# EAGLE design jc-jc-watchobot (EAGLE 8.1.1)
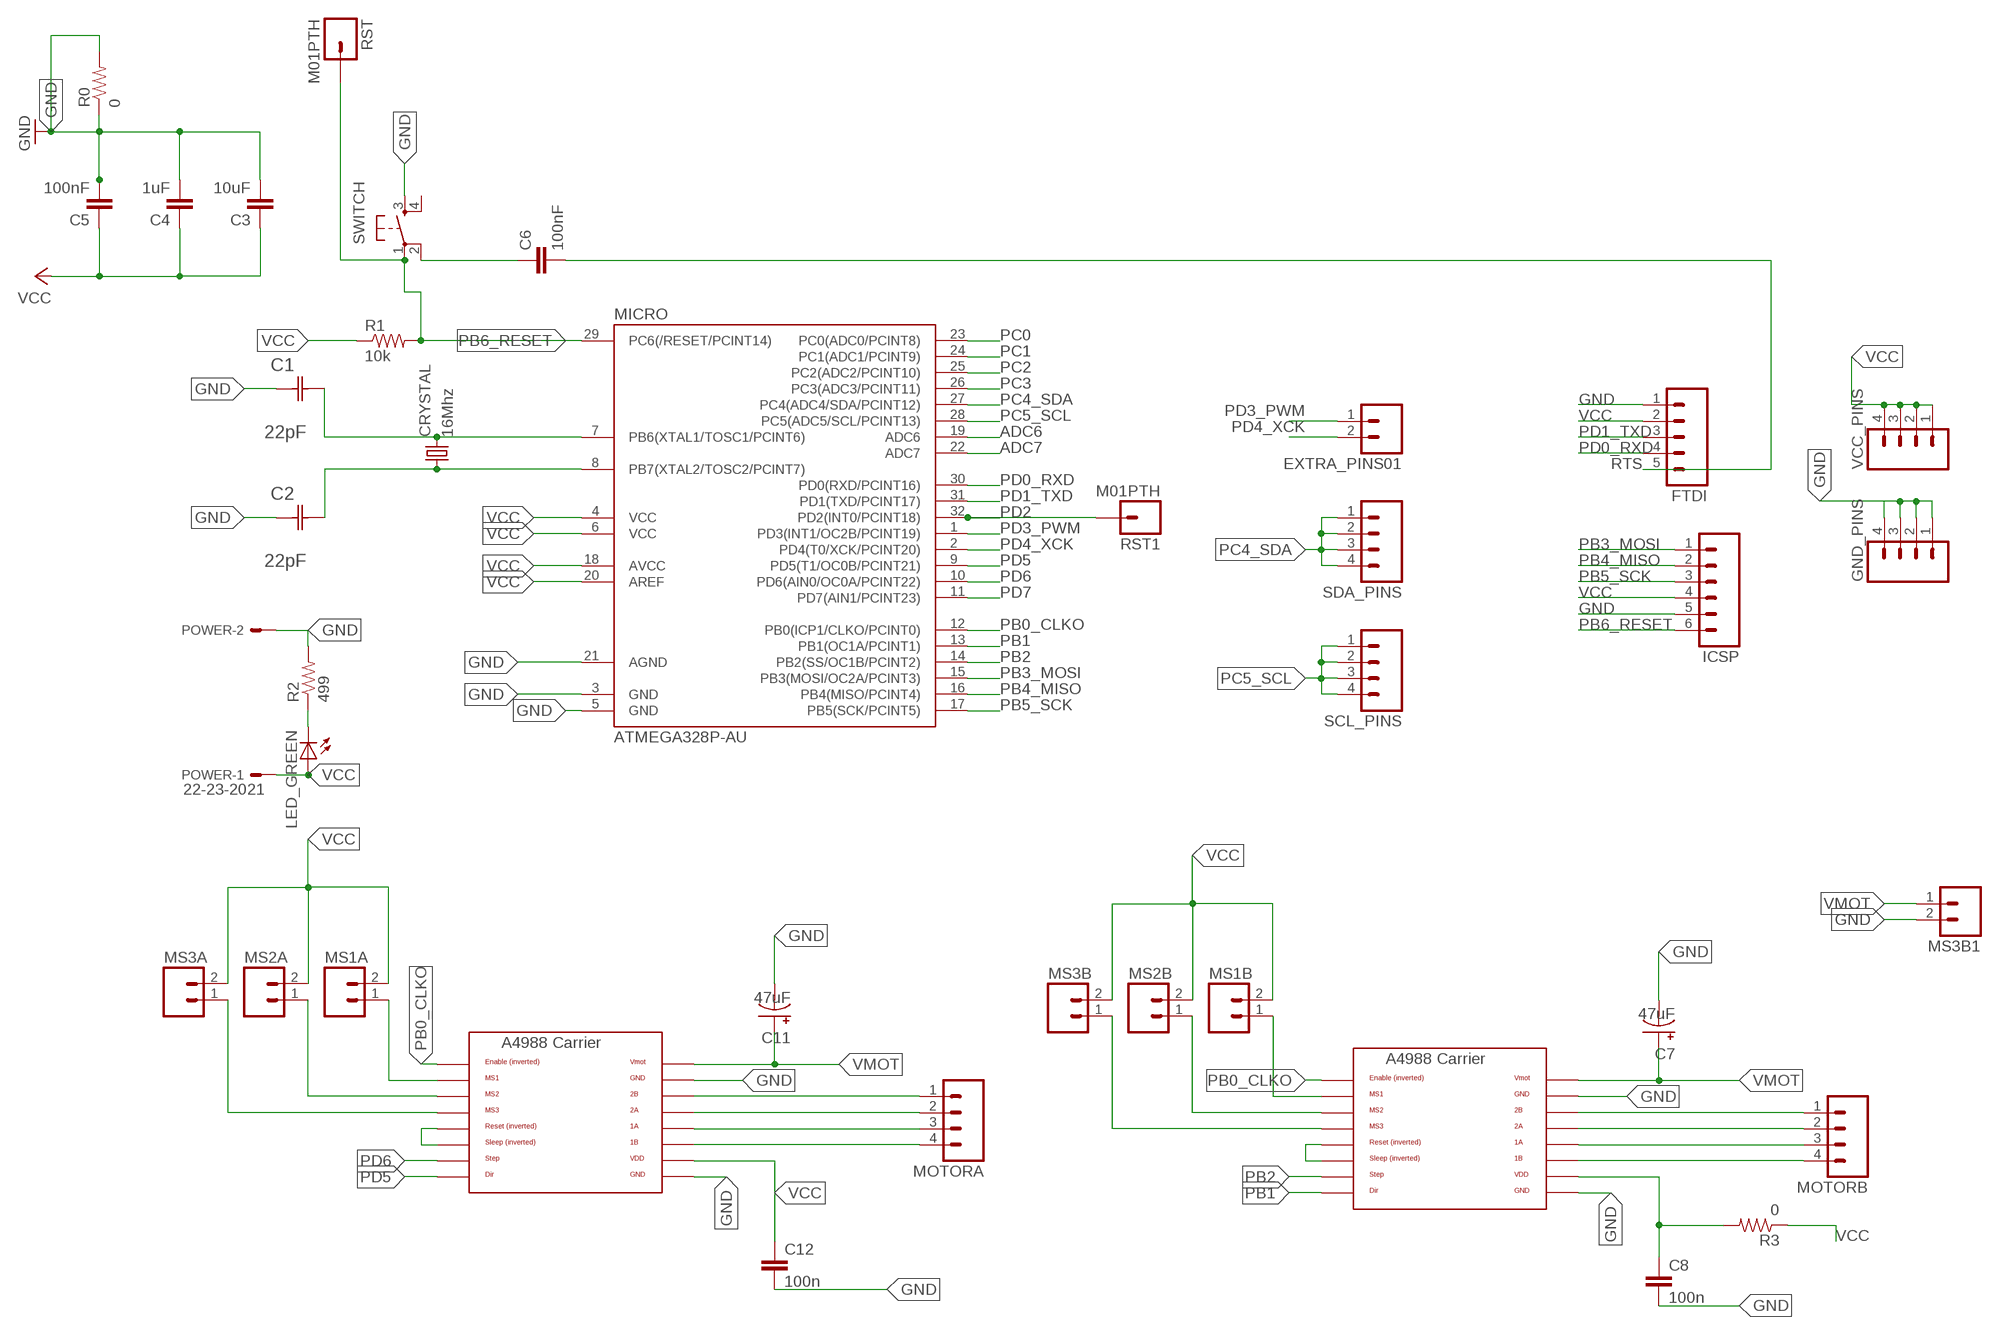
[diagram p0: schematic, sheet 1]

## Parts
C1  22pF  0612ZC225MAT2A  [CAPC3216X178N]
C2  22pF  0612ZC225MAT2A  [CAPC3216X178N]
C3  10uF  CAP1206  [1206]
C4  1uF  CAP1206  [1206]
C5  100nF  CAP1206  [1206]
C6  100nF  CAP1206  [1206]
C7  47uF  MCGPR50V107M8X11  [MCGPR50V107M8X11]
C8  100n  CAP1206  [1206]
C11  47uF  MCGPR50V107M8X11  [MCGPR50V107M8X11]
C12  100n  CAP1206  [1206]
CRYSTAL  16Mhz  CSM-7X-DU  [CSM-7X-DU]
EXTRA_PINS01  M02  [02P]
FTDI  M05  [05P]
GND_PINS  M04  [04P]
ICSP  M06  [06P]
LED_GREEN  LED1206  [1206]
MICRO  ATMEGA328P-AU  ATMEGA48/88/168-AU  [TQFP32-08]
MOTORA  M04  [04P]
MOTORA_CARRIER  A4988BREAKOUT  [A4988BREAKOUT]
MOTORB  M04  [04P]
MOTORB_CARRIER  A4988BREAKOUT  [A4988BREAKOUT]
MS1A  M02  [02P]
MS1B  M02  [02P]
MS2A  M02  [02P]
MS2B  M02  [02P]
MS3A  M02  [02P]
MS3B  M02  [02P]
MS3B1  M02  [02P]
POWER  22-23-2021  [22-23-2021]
R0  0  RESISTOR1206  [1206]
R1  10k  RESISTOR1206  [1206]
R2  499  RESISTOR1206  [1206]
R3  0  RESISTOR1206  [1206]
RST  M01PTH  [1X01]
RST1  M01PTH  [1X01]
SCL_PINS  M04  [04P]
SDA_PINS  M04  [04P]
SWITCH  6MM_SWITCH6MM_SWITCH  [6MM_SWITCH]
VCC_PINS  M04  [04P]

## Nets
ADC6: MICRO.19(ADC6)
ADC7: MICRO.22(ADC7)
GND: C1.1(C1) C2.1(C1) C3.2 C4.2 C5.2 C7.- C8.2 C11.- C12.2 FTDI.1 GND_PINS.1 GND_PINS.2 GND_PINS.3 GND_PINS.4 ICSP.5 MICRO.3(GND) MICRO.5(GND) MICRO.21(AGND) MOTORA_CARRIER.GND MOTORA_CARRIER.GND@0(GND) MOTORB_CARRIER.GND MOTORB_CARRIER.GND@0(GND) MS3B1.2 POWER.2 R0.1 R0.2 R2.2 SWITCH.3(S)
N$1: MOTORB_CARRIER.MS1 MS1B.1
N$3: MOTORA_CARRIER.MS1 MS1A.1
N$4: MOTORA_CARRIER.MS2 MS2A.1
N$5: MOTORA_CARRIER.MS3 MS3A.1
N$6: MOTORA_CARRIER.RST MOTORA_CARRIER.SLP(SLEEP)
N$7: MOTORB_CARRIER.MS2 MS2B.1
N$8: MOTORB_CARRIER.MS3 MS3B.1
N$9: MOTORB_CARRIER.RST MOTORB_CARRIER.SLP(SLEEP)
N$11: MOTORA.1 MOTORA_CARRIER.2B
N$12: MOTORA.2 MOTORA_CARRIER.2A
N$13: MOTORA.3 MOTORA_CARRIER.1A
N$14: MOTORA.4 MOTORA_CARRIER.1B
N$16: MOTORB.1 MOTORB_CARRIER.2B
N$17: MOTORB.2 MOTORB_CARRIER.2A
N$18: MOTORB.3 MOTORB_CARRIER.1A
N$19: MOTORB.4 MOTORB_CARRIER.1B
N$22: C6.1 SWITCH.2(P1)
N$26: LED_GREEN.2(C) R2.1
PB0_CLKO: MICRO.12(PB0(ICP1/CLKO/PCINT0)) MOTORA_CARRIER.EN MOTORB_CARRIER.EN
PB1: MICRO.13(PB1(OC1A/PCINT1)) MOTORB_CARRIER.DIR
PB2: MICRO.14(PB2(SS/OC1B/PCINT2)) MOTORB_CARRIER.STEP
PB3_MOSI: ICSP.1 MICRO.15(PB3(MOSI/OC2A/PCINT3))
PB4_MISO: ICSP.2 MICRO.16(PB4(MISO/PCINT4))
PB5_SCK: ICSP.3 MICRO.17(PB5(SCK/PCINT5))
PB6_RESET: ICSP.6 MICRO.29(PC6(/RESET/PCINT14)) R1.2 RST.1 SWITCH.1(P)
PB6_XTAL1: C1.2(C2) CRYSTAL.2 MICRO.7(PB6(XTAL1/TOSC1/PCINT6))
PB7_XTAL2: C2.2(C2) CRYSTAL.1 MICRO.8(PB7(XTAL2/TOSC2/PCINT7))
PC0: MICRO.23(PC0(ADC0/PCINT8))
PC1: MICRO.24(PC1(ADC1/PCINT9))
PC2: MICRO.25(PC2(ADC2/PCINT10))
PC3: MICRO.26(PC3(ADC3/PCINT11))
PC4_SDA: MICRO.27(PC4(ADC4/SDA/PCINT12)) SDA_PINS.1 SDA_PINS.2 SDA_PINS.3 SDA_PINS.4
PC5_SCL: MICRO.28(PC5(ADC5/SCL/PCINT13)) SCL_PINS.1 SCL_PINS.2 SCL_PINS.3 SCL_PINS.4
PD0_RXD: FTDI.4 MICRO.30(PD0(RXD/PCINT16))
PD1_TXD: FTDI.3 MICRO.31(PD1(TXD/PCINT17))
PD2: MICRO.32(PD2(INT0/PCINT18)) RST1.1
PD3_PWM: EXTRA_PINS01.1 MICRO.1(PD3(INT1/OC2B/PCINT19))
PD4_XCK: EXTRA_PINS01.2 MICRO.2(PD4(T0/XCK/PCINT20))
PD5: MICRO.9(PD5(T1/OC0B/PCINT21)) MOTORA_CARRIER.DIR
PD6: MICRO.10(PD6(AIN0/OC0A/PCINT22)) MOTORA_CARRIER.STEP
PD7: MICRO.11(PD7(AIN1/PCINT23))
RTS: C6.2 FTDI.5
VCC: C3.1 C4.1 C5.1 C8.1 C12.1 FTDI.2 ICSP.4 LED_GREEN.1(A) MICRO.4(VCC) MICRO.6(VCC) MICRO.18(AVCC) MICRO.20(AREF) MOTORA_CARRIER.VDD MOTORB_CARRIER.VDD MS1A.2 MS1B.2 MS2A.2 MS2B.2 MS3A.2 MS3B.2 POWER.1 R1.1 R3.1 R3.2 VCC_PINS.1 VCC_PINS.2 VCC_PINS.3 VCC_PINS.4
VMOT: C7.+ C11.+ MOTORA_CARRIER.VMOT MOTORB_CARRIER.VMOT MS3B1.1
Unconnected: SWITCH.4(S1)

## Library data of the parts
C1 C2 = AVX_By_element14_Batch_1:0612ZC225MAT2A: Capacitor 1206; MPN: 0612ZC225MAT2A; OC_FARNELL: -; OC_NEWARK: 12N3209; SUPPLIER: AVX; TOLERANCE: ±20%; VALUE: 2.2µF; VOLTAGERATING: 10V
C3-C6 C8 C12 = 01_SparkFun:CAP: Capacitor
C7 C11 = Ryan:MCGPR50V107M8X11
CRYSTAL = 01_FAB_Hello:CSM-7X-DU: SMD CRYSTAL; OC_FARNELL: unknown; OC_NEWARK: unknown
EXTRA_PINS01 MS1A MS1B MS2A MS2B MS3A MS3B MS3B1 = con-amp-quick:M02: AMP QUICK CONNECTOR; OC_FARNELL: unknown; OC_NEWARK: unknown
FTDI = con-amp-quick:M05: AMP QUICK CONNECTOR; OC_FARNELL: unknown; OC_NEWARK: unknown
GND_PINS MOTORA MOTORB SCL_PINS SDA_PINS VCC_PINS = con-amp-quick:M04: AMP QUICK CONNECTOR; OC_FARNELL: unknown; OC_NEWARK: unknown
ICSP = con-amp-quick:M06: AMP QUICK CONNECTOR; OC_FARNELL: unknown; OC_NEWARK: unknown
LED_GREEN = 01_FAB_Hello:LED
MICRO = atmega8:ATMEGA48/88/168
MOTORA_CARRIER MOTORB_CARRIER = RepRapjr:A4988BREAKOUT
POWER = con-molex:22-23-2021: .100" (2.54mm) Center Header - 2 Pin; MF: MOLEX; MPN: 22-23-2021; OC_FARNELL: 1462926; OC_NEWARK: 25C3832
R0 R1-R3 = 01_SparkFun:RESISTOR: Resistor
RST RST1 = 01_SparkFun:M01: Header 1
SWITCH = 01_FAB_Hello:6MM_SWITCH: OMRON SWITCH

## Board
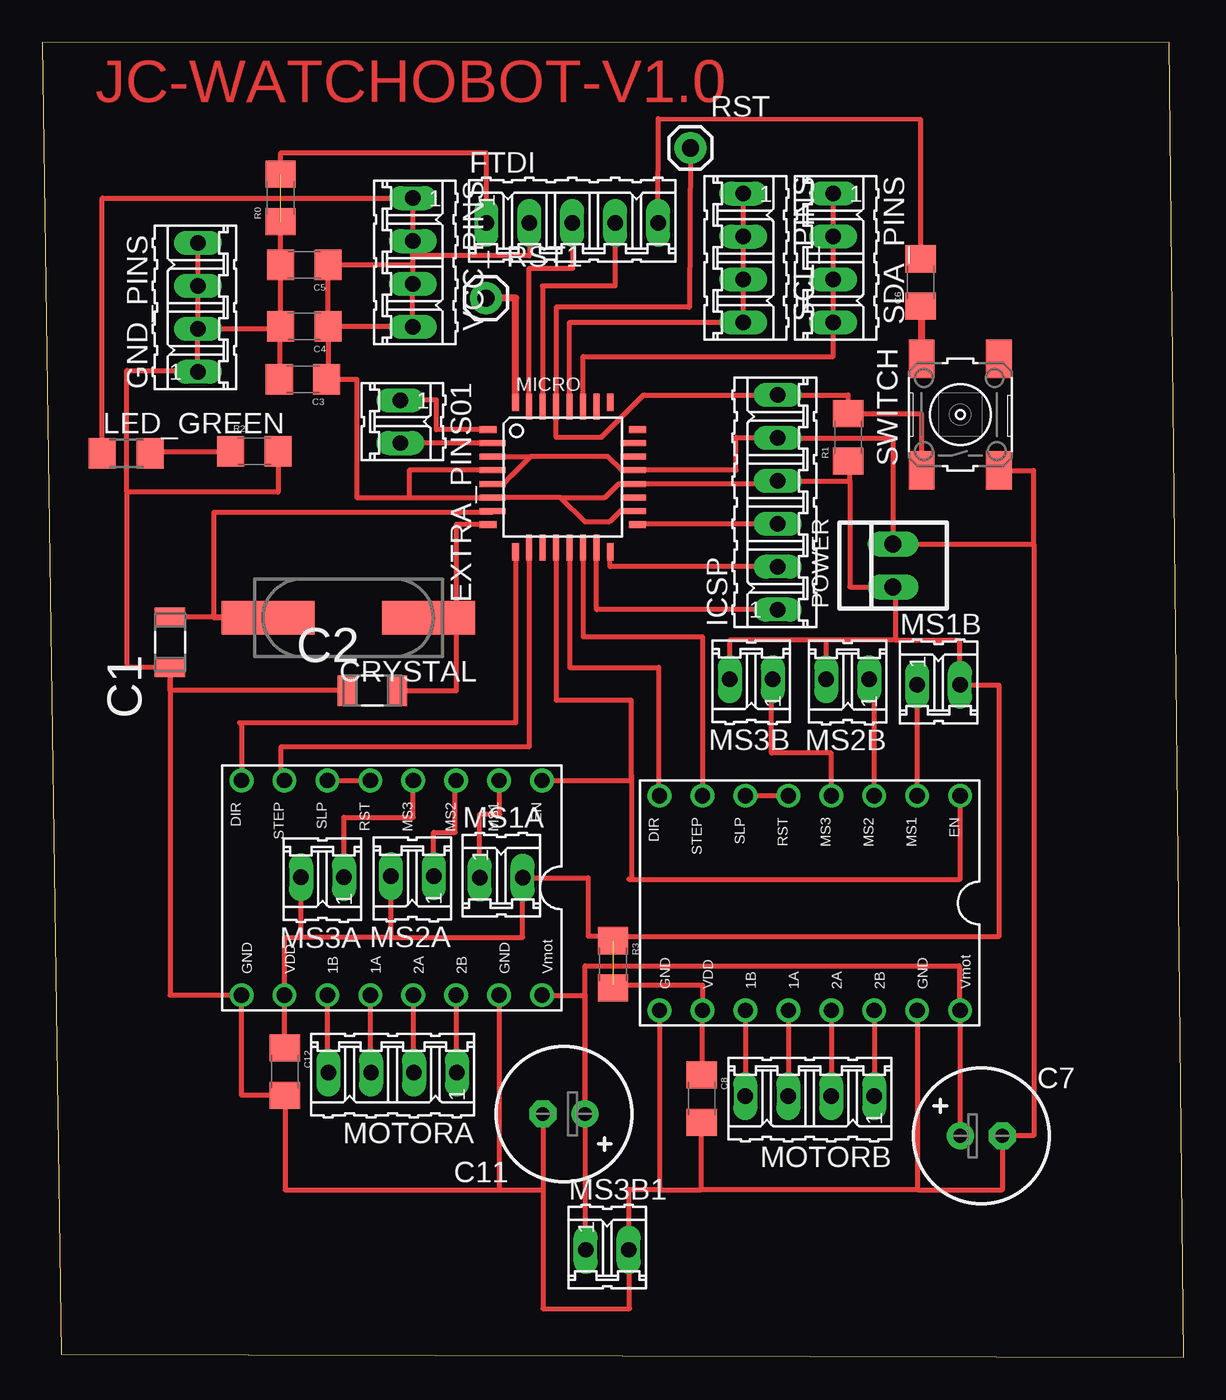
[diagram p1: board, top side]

Size 67.53 x 77.79 mm. Coordinates in mm from the lower left corner, seen from the top.
Outline: 1.11,0.17 67.53,0 66.67,77.79 0,77.78 1.11,0.17
Copper layers (1*16): Top 0.035mm / dielectric 1.5mm / Bottom 0.035mm
Design rules "default *": minimum track width 10mil, minimum drill 24mil, track to track 8mil, track to pad 8mil, pad to pad 8mil, via to via 8mil, smd to smd 8mil, copper to edge 40mil, drill to drill 8mil, minimum pad ring 10mil, minimum via ring 8mil, stop-mask expansion 4mil, vias tented up to drill 0mil, thermal gap 10mil

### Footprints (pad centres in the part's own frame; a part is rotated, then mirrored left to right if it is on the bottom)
CAPC3216X178N = smd 1.118 x 1.803: 1 -1.499,0; 2 1.499,0
1206 = smd 1.6 x 1.8: 1 -1.4,0; 2 1.4,0
MCGPR50V107M8X11 = drill 0.813 pad 1.6: + -1.25,0 | drill 0.813 pad 1.6 octagon: - 1.25,0
CSM-7X-DU = smd 5.5 x 2: 1 -4.75,0; 2 4.75,0
02P = drill 0.914 long: 1 -1.27,0; 2 1.27,0
05P = drill 0.914 long: 1 -5.08,0; 2 -2.54,0; 3 0,0; 4 2.54,0; 5 5.08,0
04P = drill 0.914 long: 1 -3.81,0; 2 -1.27,0; 3 1.27,0; 4 3.81,0
06P = drill 0.914 long: 1 -6.35,0; 2 -3.81,0; 3 -1.27,0; 4 1.27,0; 5 3.81,0; 6 6.35,0
1206' = smd 1.6 x 1.803: 1 -1.422,0; 2 1.422,0
TQFP32-08 = smd 1.016 x 0.406: 1 -4.42,2.8; 8 -4.42,-2.8; 17 4.42,-2.8; 24 4.42,2.8 | smd 1.524 x 0.356: 2 -4.166,2; 3 -4.166,1.2; 4 -4.166,0.4; 5 -4.166,-0.4; 6 -4.166,-1.2; 7 -4.166,-2; 18 4.166,-2; 19 4.166,-1.2; 20 4.166,-0.4; 21 4.166,0.4; 22 4.166,1.2; 23 4.166,2 | smd 0.406 x 1.016: 9 -2.8,-4.42; 16 2.8,-4.42; 25 2.8,4.42; 32 -2.8,4.42 | smd 0.356 x 1.524: 10 -2,-4.166; 11 -1.2,-4.166; 12 -0.4,-4.166; 13 0.4,-4.166; 14 1.2,-4.166; 15 2,-4.166; 26 2,4.166; 27 1.2,4.166; 28 0.4,4.166; 29 -0.4,4.166; 30 -1.2,4.166; 31 -2,4.166
A4988BREAKOUT = drill 0.9: 1A 8.89,1.27; 1B 11.43,1.27; 2A 6.35,1.27; 2B 3.81,1.27; DIR 16.51,-11.43; EN -1.27,-11.43; GND 16.51,1.27; GND@0 1.27,1.27; MS1 1.27,-11.43; MS2 3.81,-11.43; MS3 6.35,-11.43; RST 8.89,-11.43; SLP 11.43,-11.43; STEP 13.97,-11.43; VDD 13.97,1.27; VMOT -1.27,1.27
22-23-2021 = drill 1 long: 1 -1.27,0; 2 1.27,0
1X01 = drill 1.016 pad 1.88: 1 0,0
6MM_SWITCH = smd 2.286 x 1.524: 1 -3.302,2.286; 2 3.302,2.286; 3 -3.302,-2.286; 4 3.302,-2.286

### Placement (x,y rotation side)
C1  7.56,42.3 90 top
C2  19.53,39.44 0 top
C3  15.43,57.86 180 top
C4  15.52,60.98 180 top
C5  15.52,64.63 180 top
C6  51.98,63.58 90 top
C7  55.56,13.09 0 top
C8  39.01,15.29 270 top
C11  30.87,14.39 180 top
C12  14.36,16.9 270 top
CRYSTAL  18.1,43.75 180 top
EXTRA_PINS01  21.19,55.35 270 top
FTDI  31.36,67.11 0 top
GND_PINS  9.2,62.11 90 top
ICSP  43.5,50.58 90 top
LED_GREEN  [1206']  4.98,53.49 0 top
MICRO  30.8,52.07 0 top
MOTORA  20.72,16.85 180 top
MOTORA_CARRIER  28.3,22.69 180 top
MOTORB  45.41,15.44 180 top
MOTORB_CARRIER  53.03,21.79 180 top
MS1A  27.16,28.36 0 top
MS1B  53.03,39.79 0 top
MS2A  21.89,28.45 180 top
MS2B  47.65,40.1 180 top
MS3A  16.58,28.41 180 top
MS3B  41.95,40.12 180 top
MS3B1  33.42,6.36 0 top
POWER  50.33,46.85 90 top
R0  14.1,68.58 90 top
R1  47.68,54.42 90 top
R2  12.55,53.58 0 top
R3  33.77,23.24 270 top
RST  38.34,71.54 0 top
RST1  26.25,62.66 0 top
SCL_PINS  41.47,65.04 270 top
SDA_PINS  46.8,65.04 270 top
SWITCH  54.31,55.77 90 top
VCC_PINS  21.91,64.77 270 top

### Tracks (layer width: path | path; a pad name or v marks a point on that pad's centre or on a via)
GND  (1 unrouted)
  Top 0.305: 28.86,53.26 26.64,53.26 MICRO.3 | C2.1 7.56,39.44 C1.1 | C1.1 7.56,21.42 MOTORA_CARRIER.GND 11.79,15.5 C12.2 14.38,15.5 14.38,9.91 | 36.49,20.52 MOTORB_CARRIER.GND 36.52,9.91 36.62,9.91 | C4.2 14.12,60.84 GND_PINS.2 | C4.2 C5.2 14.12,67.18 R0.1 | GND_PINS.4 GND_PINS.3 GND_PINS.2 | GND_PINS.2 GND_PINS.1 9.2,58.37 5.01,58.37 5.01,51.17 | C1.1 5.01,40.8 5.01,51.17 | 36.62,9.91 39.01,9.91 | MOTORA_CARRIER.GND@0 27.03,9.91 | C11.- 29.62,9.91 | 51.76,9.91 56.81,9.91 C7.- 58.66,13.1 58.66,48.12 | 51.76,9.91 39.01,9.91 | MOTORB_CARRIER.GND@0 51.76,9.91 | SWITCH.3 58.66,52.46 58.66,48.12 | 58.66,48.12 POWER.2 50.33,54.39 ICSP.5 43.5,54.41 41.05,54.41 41.05,52.47 MICRO.21 34.28,52.47 33.46,53.3 28.9,53.3 28.86,53.26 | 28.86,53.26 27.76,52.16 27.76,52.15 27.28,51.67 MICRO.5 | C4.2 14.03,60.98 C3.2 | R2.2 13.96,51.17 5.01,51.17 | R0.2 14.1,71.25 26.26,71.25 FTDI.1 | 14.38,9.89 14.38,9.91 | 14.38,9.91 27.03,9.91 | 27.03,9.91 29.62,9.91 | 29.62,9.91 29.62,2.88 34.75,2.88 34.75,6.36 MS3B1.2 34.7,9.91 36.62,9.91 | 39.01,9.91 C8.2
N$1
  Top 0.305: MOTORB_CARRIER.MS1 MS1B.1 | MS1B.1
N$3
  Top 0.305: MS1A.1 25.89,32.13 27.06,32.13 27.06,34.12 MOTORA_CARRIER.MS1
N$4
  Top 0.305: MS2A.1 23.16,31.05 24.43,31.05 24.43,34.12 MOTORA_CARRIER.MS2
N$5
  Top 0.305: MS3A.1 17.85,31.95 21.94,31.95 21.94,34.12 MOTORA_CARRIER.MS3
N$6
  Top 0.305: MOTORA_CARRIER.SLP MOTORA_CARRIER.RST
N$7
  Top 0.305: MOTORB_CARRIER.MS2 49.22,40.1 MS2B.1
N$8
  Top 0.305: MOTORB_CARRIER.MS3 46.68,35.73 43.16,35.73 43.16,40.12 MS3B.1
N$9
  Top 0.305: MOTORB_CARRIER.RST MOTORB_CARRIER.SLP
N$11
  Top 0.305: MOTORA_CARRIER.2B 24.49,16.85 MOTORA.1
N$12
  Top 0.305: MOTORA_CARRIER.2A 21.95,16.85 MOTORA.2
N$13
  Top 0.305: MOTORA_CARRIER.1A 19.41,16.85 MOTORA.3
N$14
  Top 0.305: MOTORA_CARRIER.1B 16.87,16.85 MOTORA.4
N$16
  Top 0.305: MOTORB_CARRIER.2B MOTORB.1
N$17
  Top 0.305: MOTORB_CARRIER.2A MOTORB.2
N$18
  Top 0.305: MOTORB_CARRIER.1A MOTORB.3
N$19
  Top 0.305: MOTORB_CARRIER.1B MOTORB.4
N$22
  Top 0.406: C6.1 52.03,62.18 SWITCH.2
N$26
  Top 0.305: LED_GREEN.2 6.4,53.58 R2.1
PB0_CLKO
  Top 0.305: MOTORB_CARRIER.EN 54.3,28.28 34.7,28.28 34.85,28.28 34.85,34.44 | MICRO.12 30.4,38.88 34.85,38.88 34.85,34.44 | MOTORA_CARRIER.EN 34.85,34.12 34.85,34.44
PB1
  Top 0.305: MICRO.13 31.2,40.81 36.46,40.81 36.46,33.22 MOTORB_CARRIER.DIR
PB2
  Top 0.305: MICRO.14 32,42.63 39.05,42.63 39.05,33.22 MOTORB_CARRIER.STEP
PB3_MOSI
  Top 0.305: ICSP.1 32.8,44.23 MICRO.15
PB4_MISO
  Top 0.305: ICSP.2 33.6,46.77 MICRO.16
PB5_SCK
  Top 0.305: ICSP.3 35.22,49.31 MICRO.17
PB6_RESET
  Top 0.305: RST.1 38.29,62.11 30.4,62.11 MICRO.29 30.4,54.44 33.1,54.44 35.6,56.94 35.62,56.93 ICSP.6 47.68,56.93 R1.2 52.03,55.82 SWITCH.1
PB6_XTAL1
  Top 0.305: MICRO.7 26.64,50 10.17,50 10.17,43.75 CRYSTAL.2 13.35,43.8 C1.2
PB7_XTAL2
  Top 0.305: MICRO.8 24.5,49.27 24.5,43.73 | 24.5,43.73 22.85,43.73 CRYSTAL.1 | C2.2 24.5,39.44 24.5,43.73
PC4_SDA
  Top 0.305: SDA_PINS.1 SDA_PINS.2 SDA_PINS.3 SDA_PINS.4 46.81,59.2 32,59.2 MICRO.27
PC5_SCL
  Top 0.305: SCL_PINS.1 SCL_PINS.2 SCL_PINS.3 SCL_PINS.4 31.2,61.23 MICRO.28
PD0_RXD
  Top 0.305: FTDI.4 33.9,63.38 29.59,63.38 29.59,56.24 MICRO.30
PD1_TXD
  Top 0.305: MICRO.31 28.8,64.42 31.39,64.42 31.39,67.11 FTDI.3
PD2
  Top 0.406: MICRO.32 28,62.66 RST1.1
PD3_PWM
  Top 0.305: MICRO.1 23.32,54.87 23.32,56.63 21.19,56.63 EXTRA_PINS01.1
PD4_XCK
  Top 0.305: MICRO.2 EXTRA_PINS01.2
PD5
  Top 0.305: MICRO.9 28,37.53 11.66,37.53 11.79,37.53 MOTORA_CARRIER.DIR
PD6
  Top 0.305: MICRO.10 28.8,36.13 14.15,36.13 14.15,34.12 MOTORA_CARRIER.STEP
RTS
  Top 0.305: FTDI.5 36.45,73.27 51.96,73.23 51.96,64.98 C6.2
VCC  (1 unrouted)
  Top 0.305: C4.1 21.91,60.98 VCC_PINS.4 VCC_PINS.3 21.91,64.63 | 21.91,65.17 VCC_PINS.2 VCC_PINS.1 3.55,68.58 LED_GREEN.1 | 21.91,65.17 21.91,64.63 | C4.1 C5.1 21.91,64.63 | C4.1 17.09,60.98 | 26.64,50.84 MICRO.6 | 21.71,50.87 MICRO.6 | 21.71,50.87 18.61,50.87 18.61,57.86 C3.1 16.92,57.86 C4.1 | MICRO.4 21.71,52.47 21.71,50.87 | MS3B.2 40.68,42.42 46.37,42.42 | 46.37,42.42 46.37,40.1 | 50.48,42.42 54.3,42.42 MS1B.2 54.3,39.74 56.61,39.74 56.61,24.91 33.77,24.91 | 50.48,42.42 46.37,42.42 | 15.31,24.85 MS3A.2 | 20.62,24.85 15.31,24.85 | 20.62,24.85 28.43,24.85 MS1A.2 32.31,28.36 32.31,24.91 33.77,24.91 | MS2A.2 20.62,24.85 | 50.48,42.42 50.48,45.58 POWER.1 47.77,45.58 47.77,51.85 | 34.97,50.12 MICRO.18 34.2,50.07 33.55,49.42 32.1,49.42 30.65,50.87 | 30.65,50.87 33.3,50.87 34.1,51.67 MICRO.20 43.5,51.67 ICSP.4 47.77,51.85 | 30.65,50.87 MICRO.6 | R1.1 47.77,53.02 47.77,51.85 | FTDI.2 28.82,65.17 21.91,65.17 | C8.1 39.06,16.69 MOTORB_CARRIER.VDD 39.06,22.02 33.77,22.02 R3.2 | C12.1 14.33,18.3 MOTORA_CARRIER.VDD 14.33,24.85 15.31,24.85 | 33.77,24.91 R3.1 33.77,24.91
  Top 0.406: 46.37,40.1 MS2B.2
VMOT
  Top 0.305: MOTORA_CARRIER.VMOT 32.12,21.42 C11.+ | C7.+ MOTORB_CARRIER.VMOT 54.25,20.52 54.25,23.16 32.12,23.16 C11.+ | MS3B1.1 32.16,14.39 C11.+

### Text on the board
Top: JC-WATCHOBOT-V1.0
